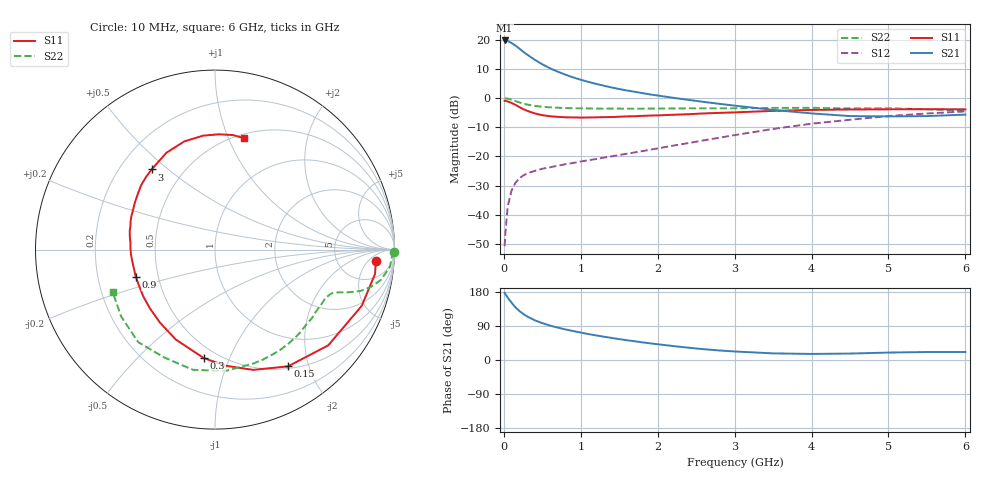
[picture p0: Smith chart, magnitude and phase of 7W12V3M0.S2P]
! Infineon Technologies  Discrete & RF Semiconductors
! BFS17W
! Si NPN RF Bipolar Junction Transistor in SOT323
! VCE = 12 V  IC = 3 mA
! Common Emitter S-Parameters:  August  1999
# GHz  S  MA  R  50
!  f  S11  S21  S12  S22
! GHz  MAG  ANG  MAG  ANG  MAG  ANG  MAG  ANG
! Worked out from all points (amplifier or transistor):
!   36 points, 10 MHz to 6 GHz, reference 50 ohm
!   highest |S21| = 19.8 dB at 10 MHz (marker M1)
!   |S21| within 3 dB of that: start of sweep to 212.5 MHz
!   unconditionally stable (mu >= 1): 754 MHz to 2.414 GHz; 5.185 GHz to end of sweep
!   at 250 MHz: K = 0.44, MSG = 21.3 dB, |S12| = -26.6 dB
!   at 1.4 GHz: K = 1.22, MAG = 9.0 dB, |S12| = -20.0 dB
!   at 6 GHz: K = 1.06, MAG = -2.0 dB, |S12| = -4.6 dB
!   S11 on the Smith chart (normalised r, x): 10 MHz: 13, -9; 150 MHz: 0.53, -1.68; 300 MHz: 0.42, -0.81; 900 MHz: 0.37, -0.15; 3 GHz: 0.33, +0.44; 6 GHz: 0.54, +1.14
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0.01  0.898 -4.2  9.725 177.3  0.0029 79.7  0.9984 -0.7
0.02  0.9021 -8.6  9.724 173.8  0.0048 86.6  0.9864 -2.3
0.05  0.8757 -20.9  9.477 164.7  0.0138 81.3  0.9795 -5.6
0.1  0.8264 -40.2  8.814 151.3  0.026 70.4  0.9396 -10.4
0.15  0.7672 -58.0  7.954 139.2  0.0353 61.1  0.8902 -13.6
0.2  0.703 -72.4  7.101 129.7  0.0419 57.0  0.8449 -15.8
0.25  0.6497 -84.8  6.275 121.9  0.047 52.3  0.8061 -17.0
0.3  0.608 -95.8  5.606 115.3  0.051 50.4  0.7771 -17.8
0.4  0.5468 -113.5  4.55 105.0  0.0566 47.6  0.7347 -18.9
0.5  0.5097 -126.9  3.799 97.3  0.0616 47.1  0.7109 -19.7
0.6  0.4886 -137.8  3.243 90.9  0.0652 48.5  0.6939 -20.6
0.7  0.4776 -146.6  2.839 85.5  0.0693 49.7  0.6839 -21.8
0.9  0.4671 -160.8  2.267 76.4  0.0772 52.9  0.6696 -24.6
1.1  0.4655 -171.9  1.895 68.4  0.0862 56.3  0.6647 -28.0
1.3  0.4716 178.8  1.632 61.5  0.0955 59.4  0.6598 -31.8
1.6  0.4865 167.6  1.35 52.1  0.1116 63.8  0.6586 -37.8
2.2  0.5176 149.6  1.013 36.8  0.1531 70.5  0.6647 -51.4
3  0.5694 128.3  0.743 22.5  0.2321 72.8  0.6699 -71.2
3.5  0.6037 116.6  0.628 17.5  0.2961 70.3  0.6786 -85.0
4.5  0.6382 96.0  0.492 17.0  0.4257 59.1  0.6642 -115.3
5.5  0.6459 81.1  0.492 21.1  0.5449 45.3  0.6423 -144.5
6  0.6415 75.4  0.521 21.1  0.5917 38.6  0.6168 -157.7
